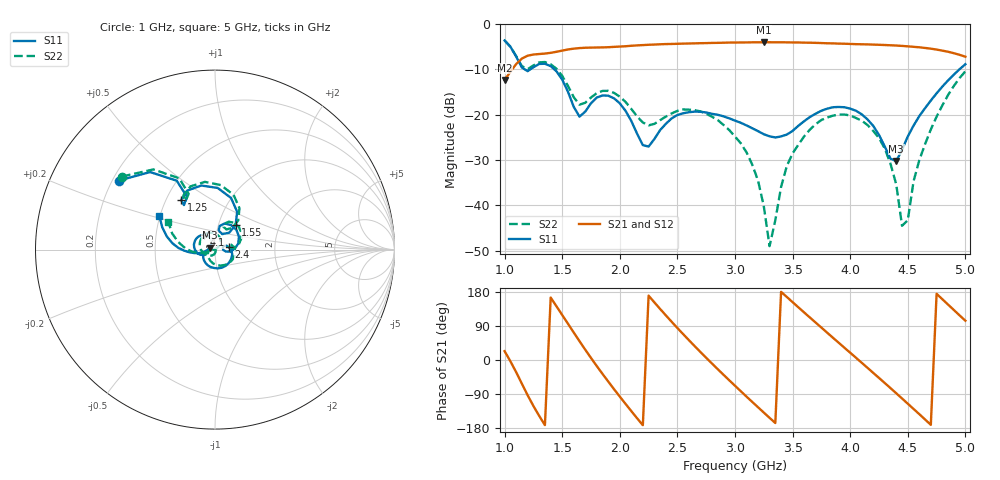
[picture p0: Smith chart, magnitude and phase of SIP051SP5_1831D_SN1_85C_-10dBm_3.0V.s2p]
# GHz  S  dB  R  50
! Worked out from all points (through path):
!   81 points, 1 GHz to 5 GHz, reference 50 ohm
!   highest |S21| = -4.01 dB at 3.25 GHz (marker M1); lowest = -12.3 dB at 1 GHz (marker M2)
!   lowest |S11| = -30.2 dB at 4.4 GHz (marker M3), VSWR 1.06, Z = 47.1 + j0.938 ohm
!   |S11| at or under -10 dB: 1.176 GHz to 1.222 GHz (46.75 MHz wide, 3.9 % of centre); 1.432 GHz to 4.948 GHz (3.516 GHz wide, 110 % of centre)
!   |S22| runs from -49.0 to -3.6 dB; largest |S21 - S12| = 0.0034
!   S11 on the Smith chart (normalised r, x): 1 GHz: 0.23, +0.31; 1.25 GHz: 0.60, +0.37; 1.55 GHz: 1.21, +0.34; 2.4 GHz: 1.17, +0.03; 4.1 GHz: 0.88, +0.15; 5 GHz: 0.50, +0.21
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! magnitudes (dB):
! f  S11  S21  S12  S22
! 1 GHz  -3.6  -12.3  -12.3  -3.6
! 1.25 GHz  -9.5  -6.7  -6.7  -9.1
! 1.55 GHz  -14.9  -5.6  -5.6  -13.6
! 1.7 GHz  -19.3  -5.2  -5.2  -17.4
! 1.9 GHz  -15.8  -5.1  -5.1  -14.7
! 2.2 GHz  -26.7  -4.6  -4.6  -21.7
! 2.35 GHz  -23.4  -4.5  -4.5  -21.2
! 2.4 GHz  -22.0  -4.4  -4.4  -20.4
! 2.7 GHz  -19.3  -4.2  -4.2  -19.2
! 3 GHz  -21.3  -4.1  -4.1  -24.8
! 3.15 GHz  -23.0  -4.0  -4.0  -31.0
! 3.25 GHz  -24.3  -4.0  -4.0  -40.2
! 3.3 GHz  -24.7  -4.0  -4.0  -49.0
! 3.45 GHz  -24.4  -4.0  -4.0  -31.3
! 3.7 GHz  -19.8  -4.1  -4.1  -22.1
! 4.1 GHz  -19.9  -4.5  -4.4  -21.3
! 4.35 GHz  -29.7  -4.7  -4.7  -30.8
! 4.4 GHz  -30.2  -4.7  -4.7  -35.4
! 4.45 GHz  -27.7  -4.8  -4.8  -44.5
! 4.5 GHz  -24.8  -4.9  -4.9  -43.2
! 4.65 GHz  -18.5  -5.3  -5.3  -26.5
! 5 GHz  -8.9  -7.2  -7.2  -10.4
